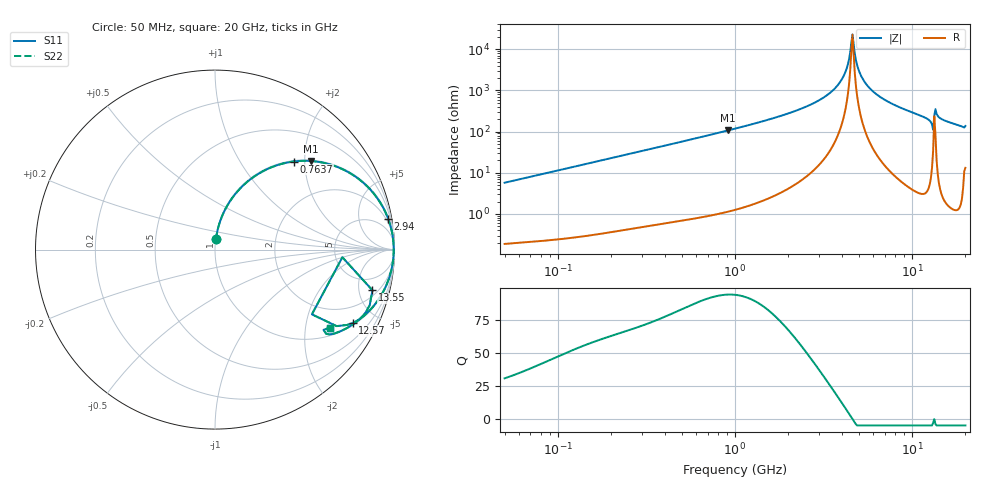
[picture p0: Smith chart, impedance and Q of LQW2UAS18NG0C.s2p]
!Murata Part Number: LQW2UAS18NG0C
!These Parameters are Measured in Series Mode Connection
!  o--[Z]--o
!Port1  Port2
!  o-------o
!Freq. Start=50[MHz] Stop=20[GHz], 401[Steps]
# Hz S RI R 50
!Freq.(Hz) S11(Real) S11(Imag) S21(Real) S21(Imag) S12(Real) S12(Imag) S22(Real) S22(Imag)
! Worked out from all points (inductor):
!   401 points, 50 MHz to 20 GHz, reference 50 ohm
!   read as one part in series: L = 18.2 nH near 51.52 MHz
!   highest Q = 94 at 914 MHz (marker M1), where L = 18.6 nH
!   self-resonance near 4.54 GHz
!   S11 on the Smith chart (normalised r, x): 50 MHz: 1.00, +0.11; 763.7 MHz: 1.02, +1.77; 2.94 GHz: 1, +11; 12.57 GHz: 1.10, -3.70; 13.55 GHz: 2.70, -6.82; 20 GHz: 1.26, -2.73
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5e7  0.00513 0.057  0.9949 -0.057  0.9949 -0.057  0.00513 0.057
1.364002e8  0.0261 0.1507  0.9739 -0.1507  0.9739 -0.1507  0.0261 0.1507
3.721004e8  0.1548 0.3551  0.8452 -0.3551  0.8452 -0.3551  0.1548 0.3551
7.636728e8  0.4385 0.4908  0.5615 -0.4908  0.5615 -0.4908  0.4385 0.4908
9.140482e8  0.5329 0.4936  0.4671 -0.4936  0.4671 -0.4936  0.5329 0.4936
1e9  0.5806 0.4882  0.4194 -0.4882  0.4194 -0.4882  0.5806 0.4882
2.728004e9  0.9528 0.2011  0.0472 -0.2011  0.0472 -0.2011  0.9528 0.2011
2.940159e9  0.9645 0.1724  0.0355 -0.1724  0.0355 -0.1724  0.9645 0.1724
3.967106e9  0.9923 0.0572  0.00771 -0.0572  0.00771 -0.0572  0.9923 0.0572
4.275624e9  0.9948 0.0284  0.00518 -0.0284  0.00518 -0.0284  0.9948 0.0284
4.472136e9  0.9955 0.0111  0.00447 -0.0111  0.00447 -0.0111  0.9955 0.0111
4.608136e9  0.9957 -0.000456  0.00433 0.000456  0.00433 0.000456  0.9957 -0.000456
4.748272e9  0.9955 -0.012  0.00447 0.012  0.00447 0.012  0.9955 -0.012
4.966507e9  0.9948 -0.0293  0.00517 0.0293  0.00517 0.0293  0.9948 -0.0293
5.352748e9  0.9923 -0.0582  0.0077 0.0582  0.0077 0.0582  0.9923 -0.0582
7.442007e9  0.9595 -0.1866  0.0405 0.1866  0.0405 0.1866  0.9595 -0.1866
1.257102e10  0.7674 -0.4088  0.2326 0.4088  0.2326 0.4088  0.7674 -0.4088
1.295331e10  0.6777 -0.4263  0.3223 0.4263  0.3223 0.4263  0.6777 -0.4263
1.354865e10  0.8772 -0.2265  0.1228 0.2265  0.1228 0.2265  0.8772 -0.2265
1.396067e10  0.8428 -0.3451  0.1572 0.3451  0.1572 0.3451  0.8428 -0.3451
1.504638e10  0.7823 -0.4068  0.2177 0.4068  0.2177 0.4068  0.7823 -0.4068
2e10  0.6394 -0.4342  0.3606 0.4342  0.3606 0.4342  0.6394 -0.4342
